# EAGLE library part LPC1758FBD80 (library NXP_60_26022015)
32-bit ARM Cortex-M3 MCU; up to 512 kB flash and 64 kB SRAM with Ethernet, USB 2.0 Host/Device/OTG, CAN The LPC1759/58/56/54/52/51 are ARM Cortex-M3 based microcontrollers for embedded applications featuring a high level of integration and low power consumption. The ARM Cortex-M3 is a next generation core that offers system enhancements such as enhanced debug features and a higher level of support block integration. The LPC1758/56/57/54/52/51 operate at CPU frequencies of up to 100 MHz. The LPC1759 operates at CPU frequencies of up to 120 MHz. The ARM Cortex-M3 CPU incorporates a 3-stage pipeline and uses a Harvard architecture with separate local instruction and data buses as well as a third bus for peripherals. The ARM Cortex-M3 CPU also includes an internal prefetch unit that supports speculative branching. The peripheral complement of the LPC1759/58/56/54/52/51 includes up to 512 kB of flash memory, up to 64 kB of data memory, Ethernet MAC, USB Device/Host/OTG interface, 8-channel general purpose DMA controller, 4 UARTs, 2 CAN channels, 2 SSP controllers, SPI interface, 2 I 2 C-bus interfaces, 2-input plus 2-output I 2 S-bus interface, 6 channel 12-bit ADC, 10-bit DAC, motor control PWM, Quadrature Encoder interface, 4 general purpose timers, 6-output general purpose PWM, ultra-low power Real-Time Clock (RTC) with separate battery supply, and up to 52 general purpose I/O pins. AAL Eindhoven MK
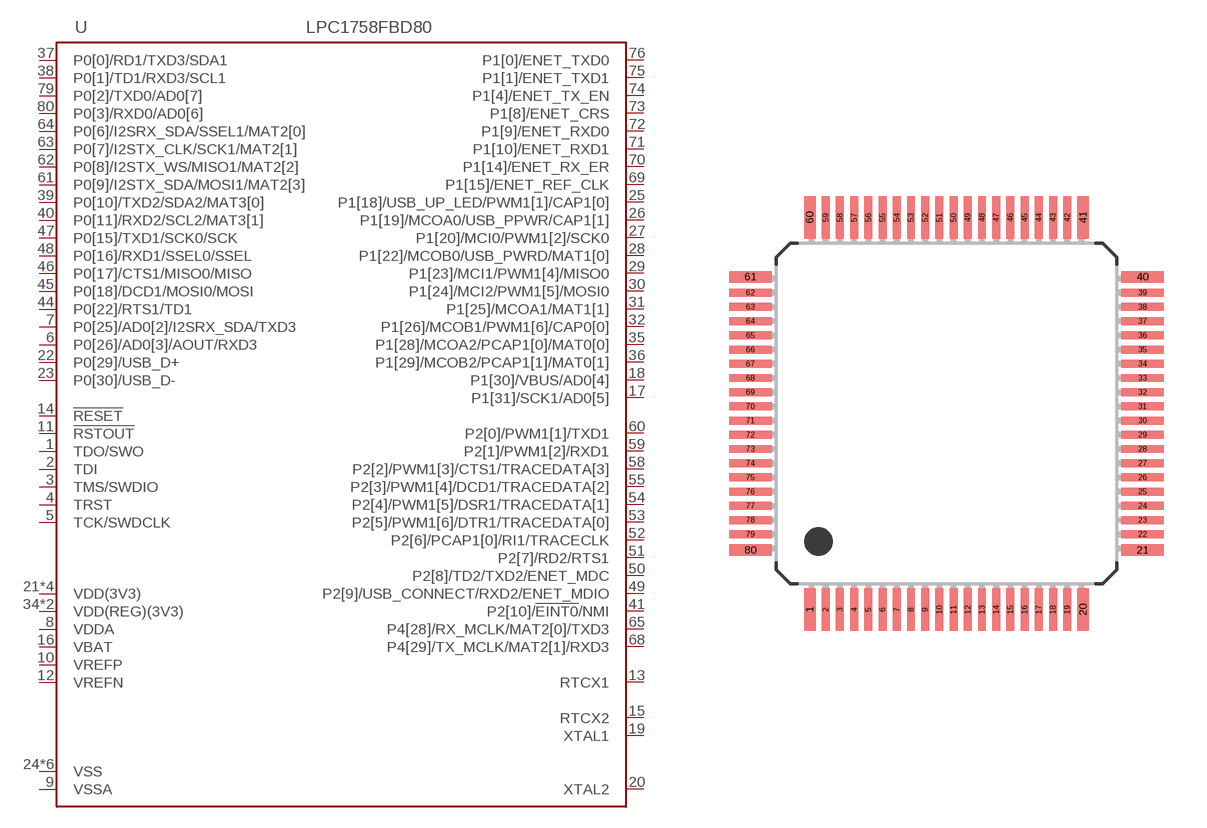
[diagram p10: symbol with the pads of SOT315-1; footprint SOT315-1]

Designator prefix U

## LPC1758FBD80 (CAN: 2; DAC: yes; ETH: yes; FLASH: 512kB; I2S: yes; MHZ: 100; SRAM: 32kB; SRAM0: 16kB; SRAM1: 16kB; USB: D/H/OTG)  [SOT315-1]
1  TDO/SWO  out
2  TDI  in
3  TMS/SWDIO
4  TRST
5  TCK/SWDCLK
6  P0[26]/AD0[3]/AOUT/RXD3
7  P0[25]/AD0[2]/I2SRX_SDA/TXD3
8  VDDA  pwr
9  VSSA  pwr
10  VREFP  in
11  !RSTOUT!  out
12  VREFN  in
13  RTCX1  in
14  !RESET!  in
15  RTCX2  out
16  VBAT  pwr
17  P1[31]/SCK1/AD0[5]
18  P1[30]/VBUS/AD0[4]
19  XTAL1  in
20  XTAL2  out
21  VDD(3V3)  pwr
22  P0[29]/USB_D+
23  P0[30]/USB_D-
24  VSS  pwr
25  P1[18]/USB_UP_LED/PWM1[1]/CAP1[0]
26  P1[19]/MCOA0/USB_PPWR/CAP1[1]
27  P1[20]/MCI0/PWM1[2]/SCK0
28  P1[22]/MCOB0/USB_PWRD/MAT1[0]
29  P1[23]/MCI1/PWM1[4]/MISO0
30  P1[24]/MCI2/PWM1[5]/MOSI0
31  P1[25]/MCOA1/MAT1[1]
32  P1[26]/MCOB1/PWM1[6]/CAP0[0]
33  VSS  pwr
34  VDD(REG)(3V3)  pwr
35  P1[28]/MCOA2/PCAP1[0]/MAT0[0]
36  P1[29]/MCOB2/PCAP1[1]/MAT0[1]
37  P0[0]/RD1/TXD3/SDA1
38  P0[1]/TD1/RXD3/SCL1
39  P0[10]/TXD2/SDA2/MAT3[0]
40  P0[11]/RXD2/SCL2/MAT3[1]
41  P2[10]/!EINT0!/NMI
42  VDD(3V3)  pwr
43  VSS  pwr
44  P0[22]/RTS1/TD1
45  P0[18]/DCD1/MOSI0/MOSI
46  P0[17]/CTS1/MISO0/MISO
47  P0[15]/TXD1/SCK0/SCK
48  P0[16]/RXD1/SSEL0/SSEL
49  P2[9]/USB_CONNECT/RXD2/ENET_MDIO
50  P2[8]/TD2/TXD2/ENET_MDC
51  P2[7]/RD2/RTS1
52  P2[6]/PCAP1[0]/RI1/TRACECLK
53  P2[5]/PWM1[6]/DTR1/TRACEDATA[0]
54  P2[4]/PWM1[5]/DSR1/TRACEDATA[1]
55  P2[3]/PWM1[4]/DCD1/TRACEDATA[2]
56  VDD(3V3)  pwr
57  VSS  pwr
58  P2[2]/PWM1[3]/CTS1/TRACEDATA[3]
59  P2[1]/PWM1[2]/RXD1
60  P2[0]/PWM1[1]/TXD1
61  P0[9]/I2STX_SDA/MOSI1/MAT2[3]
62  P0[8]/I2STX_WS/MISO1/MAT2[2]
63  P0[7]/I2STX_CLK/SCK1/MAT2[1]
64  P0[6]/I2SRX_SDA/SSEL1/MAT2[0]
65  P4[28]/RX_MCLK/MAT2[0]/TXD3
66  VSS  pwr
67  VDD(REG)(3V3)  pwr
68  P4[29]/TX_MCLK/MAT2[1]/RXD3
69  P1[15]/ENET_REF_CLK
70  P1[14]/ENET_RX_ER
71  P1[10]/ENET_RXD1
72  P1[9]/ENET_RXD0
73  P1[8]/ENET_CRS
74  P1[4]/ENET_TX_EN
75  P1[1]/ENET_TXD1
76  P1[0]/ENET_TXD0
77  VDD(3V3)  pwr
78  VSS  pwr
79  P0[2]/TXD0/AD0[7]
80  P0[3]/RXD0/AD0[6]

## Footprint SOT315-1 (pad centres in mm)
SOT315-1 LQFP80: plastic low profile quad flat package; 80 leads; body 12 x 12 x 1.4 mm JEDEC: MS-026 IEC: 136E15
smd 0.4 x 1.5: 1 -4.81,-6.9; 20 4.81,-6.9; 41 4.81,6.9; 60 -4.81,6.9
smd 0.28 x 1.5: 2 -4.25,-6.9; 3 -3.75,-6.9; 4 -3.25,-6.9; 5 -2.75,-6.9; 6 -2.25,-6.9; 7 -1.75,-6.9; 8 -1.25,-6.9; 9 -0.75,-6.9; 10 -0.25,-6.9; 11 0.25,-6.9; 12 0.75,-6.9; 13 1.25,-6.9; 14 1.75,-6.9; 15 2.25,-6.9; 16 2.75,-6.9; 17 3.25,-6.9; 18 3.75,-6.9; 19 4.25,-6.9; 42 4.25,6.9; 43 3.75,6.9; 44 3.25,6.9; 45 2.75,6.9; 46 2.25,6.9; 47 1.75,6.9; 48 1.25,6.9; 49 0.75,6.9; 50 0.25,6.9; 51 -0.25,6.9; 52 -0.75,6.9; 53 -1.25,6.9; 54 -1.75,6.9; 55 -2.25,6.9; 56 -2.75,6.9; 57 -3.25,6.9; 58 -3.75,6.9; 59 -4.25,6.9
smd 1.5 x 0.4: 21 6.9,-4.81; 40 6.9,4.81; 61 -6.9,4.81; 80 -6.9,-4.81
smd 1.5 x 0.28: 22 6.9,-4.25; 23 6.9,-3.75; 24 6.9,-3.25; 25 6.9,-2.75; 26 6.9,-2.25; 27 6.9,-1.75; 28 6.9,-1.25; 29 6.9,-0.75; 30 6.9,-0.25; 31 6.9,0.25; 32 6.9,0.75; 33 6.9,1.25; 34 6.9,1.75; 35 6.9,2.25; 36 6.9,2.75; 37 6.9,3.25; 38 6.9,3.75; 39 6.9,4.25; 62 -6.9,4.25; 63 -6.9,3.75; 64 -6.9,3.25; 65 -6.9,2.75; 66 -6.9,2.25; 67 -6.9,1.75; 68 -6.9,1.25; 69 -6.9,0.75; 70 -6.9,0.25; 71 -6.9,-0.25; 72 -6.9,-0.75; 73 -6.9,-1.25; 74 -6.9,-1.75; 75 -6.9,-2.25; 76 -6.9,-2.75; 77 -6.9,-3.25; 78 -6.9,-3.75; 79 -6.9,-4.25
